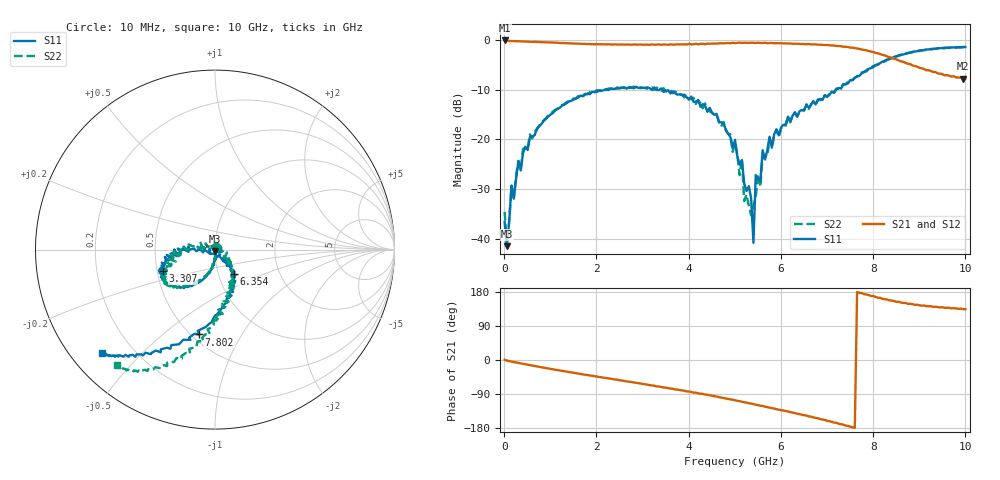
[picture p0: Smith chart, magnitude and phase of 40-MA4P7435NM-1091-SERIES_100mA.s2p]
!Agilent Technologies,E8364C,MY48140145,A.09.42.15
!Agilent E8364C: A.09.42.15
!Date: Wednesday, December 02, 2020 13:42:42
!Correction: S11(Full 2 Port(1,2))
!S21(Full 2 Port(1,2))
!S12(Full 2 Port(1,2))
!S22(Full 2 Port(1,2))
!S2P File: Measurements: S11, S21, S12, S22:
# Hz S  dB  R 50
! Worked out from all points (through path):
!   201 points, 10 MHz to 10 GHz, reference 50 ohm
!   highest |S21| = -0.09 dB at 10 MHz (marker M1); lowest = -7.8 dB at 9.95 GHz (marker M2)
!   group delay of S21, straight-line fit = 66.2 ps
!   lowest |S11| = -41.5 dB at 59.95 MHz (marker M3), VSWR 1.02, Z = 50.1 - j0.837 ohm
!   |S11| at or under -10 dB: start of sweep to 2.175 GHz; 3.301 GHz to 3.366 GHz (65.32 MHz wide, 1.96 % of centre); 3.426 GHz to 7.198 GHz (3.772 GHz wide, 71 % of centre)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
!   |S22| runs from -41.0 to -1.5 dB; largest |S21 - S12| = 0.027
!   S11 on the Smith chart (normalised r, x): 10 MHz: 1.02, +0.02; 3.307 GHz: 0.54, -0.14; 6.354 GHz: 1.18, -0.33; 7.802 GHz: 0.55, -0.67; 10 GHz: 0.09, -0.39
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1e7  -36.56 41.2  -0.09 0.9  -0.12 -0.7  -34.56 66.3
5.995e7  -41.45 -80.7  -0.16 -1.5  -0.16 -1.7  -40.97 -86.8
1.5985e8  -29.33 -83.7  -0.20 -4.2  -0.19 -4.2  -29.24 -81.7
2.098e8  -31.89 -82.2  -0.21 -5.4  -0.20 -5.4  -31.80 -88.2
3.097e8  -24.28 -91.3  -0.25 -7.7  -0.25 -7.8  -24.41 -89.7
5.5945e8  -19.49 -99.9  -0.35 -13.6  -0.34 -13.6  -18.99 -99.8
1.7083e9  -11.31 -130.0  -0.77 -37.9  -0.74 -37.6  -11.09 -133.0
3.3067e9  -10.06 -157.9  -0.92 -69.7  -0.93 -69.0  -9.57 -153.7
3.35665e9  -10.07 -160.9  -0.89 -70.0  -0.90 -70.5  -9.94 -151.5
4.35565e9  -13.16 -174.6  -0.84 -91.2  -0.79 -90.4  -12.76 -177.6
5.005e9  -20.06 170.7  -0.62 -106.3  -0.57 -106.3  -20.56 152.2
5.35465e9  -31.79 -83.8  -0.54 -115.0  -0.55 -115.0  -35.27 -33.0
5.4046e9  -40.78 -115.4  -0.56 -116.5  -0.53 -116.6  -33.32 57.5
5.45455e9  -27.16 -75.0  -0.59 -117.7  -0.57 -117.7  -31.62 -39.4
5.55445e9  -28.37 -56.3  -0.59 -120.6  -0.57 -120.6  -29.52 -6.9
5.6044e9  -22.15 -53.7  -0.60 -121.4  -0.61 -121.4  -23.16 -39.0
6.35365e9  -15.31 -52.9  -0.76 -141.7  -0.72 -141.6  -15.44 -58.5
6.7033e9  -12.26 -65.6  -0.88 -151.3  -0.87 -151.3  -12.53 -63.9
7.8022e9  -6.36 -100.5  -2.00 173.8  -1.93 174.5  -6.50 -96.2
8.35165e9  -3.78 -117.9  -3.45 157.4  -3.36 158.3  -3.86 -109.5
9.95005e9  -1.39 -137.1  -7.80 134.2  -7.71 135.2  -1.49 -129.9
1e10  -1.42 -137.6  -7.75 134.0  -7.75 133.9  -1.47 -130.2
